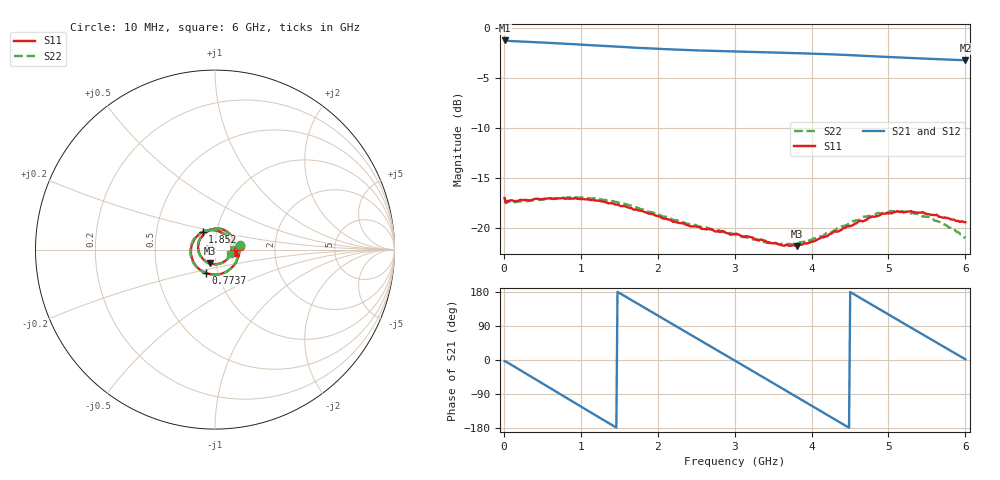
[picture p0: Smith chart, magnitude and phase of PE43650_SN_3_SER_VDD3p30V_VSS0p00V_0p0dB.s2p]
!Keysight Technologies,N5245B,MY57181451,A.13.50.07
!Date: Tuesday, May 07, 2019 07:59:43
!Correction: S11(Full 2 Port(1,2))
!S21(Full 2 Port(1,2))
!S12(Full 2 Port(1,2))
!S22(Full 2 Port(1,2))
!S2P File: Measurements: S11, S21, S12, S22:
# Hz S  dB  R 50
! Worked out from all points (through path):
!   401 points, 10 MHz to 6 GHz, reference 50 ohm
!   highest |S21| = -1.23 dB at 10 MHz (marker M1); lowest = -3.2 dB at 6 GHz (marker M2)
!   group delay of S21, straight-line fit = 332 ps
!   lowest |S11| = -21.9 dB at 3.814 GHz (marker M3), VSWR 1.18, Z = 46.7 - j7.08 ohm
!   |S11| at or under -10 dB: start of sweep to end of sweep
!   |S22| runs from -21.7 to -17.0 dB; largest |S21 - S12| = 0.0061
!   S11 on the Smith chart (normalised r, x): 10 MHz: 1.32, +0.06; 773.7 MHz: 0.88, -0.24; 1.852 GHz: 0.86, +0.17; 6 GHz: 1.23, -0.05
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1e7  -17.04 9.1  -1.23 -3.3  -1.28 -3.2  -17.06 10.2
2.1965e8  -17.22 -32.7  -1.34 -27.7  -1.39 -27.7  -17.38 -32.9
4.44275e8  -17.10 -65.2  -1.42 -55.2  -1.47 -55.2  -17.20 -65.8
7.73725e8  -17.05 -110.5  -1.55 -95.4  -1.60 -95.4  -16.99 -111.0
1.013325e9  -17.14 -141.6  -1.66 -124.4  -1.70 -124.4  -16.97 -142.2
1.432625e9  -17.63 169.0  -1.83 -174.8  -1.89 -174.8  -17.37 168.8
1.851925e9  -18.50 125.3  -2.01 135.1  -2.07 135.1  -18.32 124.6
2.01665e9  -18.88 109.5  -2.07 115.5  -2.12 115.5  -18.71 108.8
2.241275e9  -19.48 88.2  -2.15 88.8  -2.20 88.9  -19.29 87.4
2.4659e9  -19.88 66.2  -2.21 62.2  -2.27 62.2  -19.69 65.7
2.750425e9  -20.40 38.1  -2.29 28.4  -2.34 28.5  -20.26 36.5
3.005e9  -20.61 8.2  -2.34 -1.9  -2.39 -1.8  -20.68 7.5
3.45425e9  -21.55 -52.9  -2.43 -55.4  -2.47 -55.3  -21.48 -55.2
3.81365e9  -21.86 -111.0  -2.51 -98.3  -2.55 -98.2  -21.66 -113.1
4.008325e9  -21.39 -143.2  -2.55 -121.5  -2.60 -121.5  -21.17 -145.0
4.2629e9  -20.58 176.3  -2.62 -152.0  -2.68 -151.9  -20.44 174.9
4.5025e9  -19.85 141.2  -2.71 179.4  -2.76 179.5  -19.49 139.8
4.7421e9  -19.02 109.0  -2.79 150.8  -2.85 150.9  -18.83 108.2
5.01165e9  -18.56 77.1  -2.89 118.8  -2.94 119.0  -18.38 75.3
5.445925e9  -18.46 32.3  -3.04 67.3  -3.09 67.5  -18.92 28.4
5.745425e9  -19.04 7.6  -3.14 31.9  -3.19 31.9  -19.74 1.2
6e9  -19.46 -10.0  -3.21 1.8  -3.26 1.8  -21.04 -17.6
